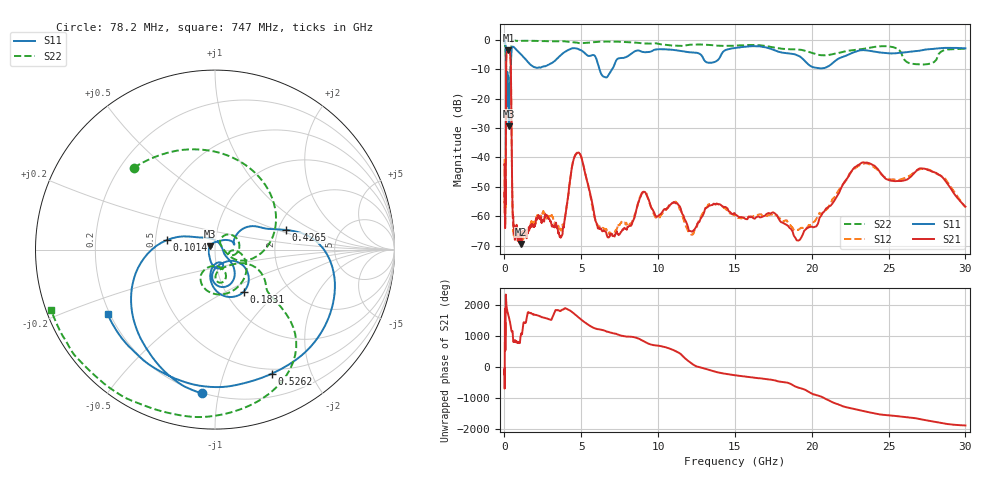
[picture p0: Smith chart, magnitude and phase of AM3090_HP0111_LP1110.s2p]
! Date/Time: Thu, Feb 28, 2019 2:01 PM
! Network Analyzer: Agilent Technologies E8364B Rev: A.07.50.67
! Sweep from 0.010 to 30.000 GHz, 1601 Points, Sweep Type: LOG
! Power Supply: 5.023 V, 0.002 A
# Hz S DB R 50
!freq MagS11 AngS11 MagS21 AngS21 MagS12 AngS12 MagS22 AngS22
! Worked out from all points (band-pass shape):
!   1601 points, 10 MHz to 30 GHz, reference 50 ohm
!   highest |S21| = -3.51 dB at 259.9 MHz (marker M1); lowest = -69.5 dB at 1.087 GHz (marker M2)
!   |S21| within 3 dB of the highest: 116.5 MHz to 397.2 MHz (280.8 MHz wide, 109 % of centre)
!   lowest |S11| = -29.4 dB at 314.3 MHz (marker M3), VSWR 1.07, Z = 47.2 + j1.63 ohm
!   |S11| at or under -10 dB: 100.6 MHz to 410.4 MHz (309.8 MHz wide, 121 % of centre); 6.184 GHz to 7.01 GHz (826.4 MHz wide, 12.5 % of centre)
!   |S22| runs from -27.7 to -0.2 dB; largest |S21 - S12| = 0.013
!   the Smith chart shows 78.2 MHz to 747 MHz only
!   S11 on the Smith chart (normalised r, x): 78.2 MHz: 0.20, -0.89; 101.4 MHz: 0.57, +0.07; 183.1 MHz: 1.21, -0.62; 426.5 MHz: 2.21, +0.58; 526.2 MHz: 0.45, -1.46; 747 MHz: 0.19, -0.27
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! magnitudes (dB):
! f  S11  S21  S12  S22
! 10 MHz  -0.3  -42.4  -40.5  -0.7
! 38.04 MHz  -0.5  -60.5  -61.1  -1.6
! 78.2 MHz  -1.9  -52.4  -55.7  -3.8
! 101.4 MHz  -11.2  -18.1  -18.1  -11.8
! 109.3 MHz  -27.9  -9.0  -9.0  -26.8
! 144.7 MHz  -20.9  -4.2  -4.2  -21.2
! 183.1 MHz  -10.9  -3.7  -3.7  -12.8
! 259.9 MHz  -21.1  -3.5  -3.5  -19.1
! 314.3 MHz  -29.4  -3.9  -3.8  -15.6
! 426.5 MHz  -7.7  -12.9  -12.9  -5.8
! 526.2 MHz  -2.4  -58.4  -56.3  -0.5
! 550.5 MHz  -2.4  -60.3  -60.7  -0.4
! 747 MHz  -3.1  -65.0  -66.2  -0.3
! 1.087 GHz  -5.0  -69.5  -68.0  -0.3
! 2.084 GHz  -9.5  -61.0  -60.3  -0.3
! 3.704 GHz  -5.0  -66.8  -64.6  -0.4
! 4.781 GHz  -3.0  -38.4  -38.2  -1.0
! 6.11 GHz  -8.7  -64.0  -63.3  -0.6
! 7.926 GHz  -5.8  -64.3  -62.2  -0.7
! 19.51 GHz  -6.9  -65.0  -63.6  -3.6
! 23.48 GHz  -3.5  -41.8  -41.9  -2.9
! 30 GHz  -2.9  -56.7  -57.0  -3.0
